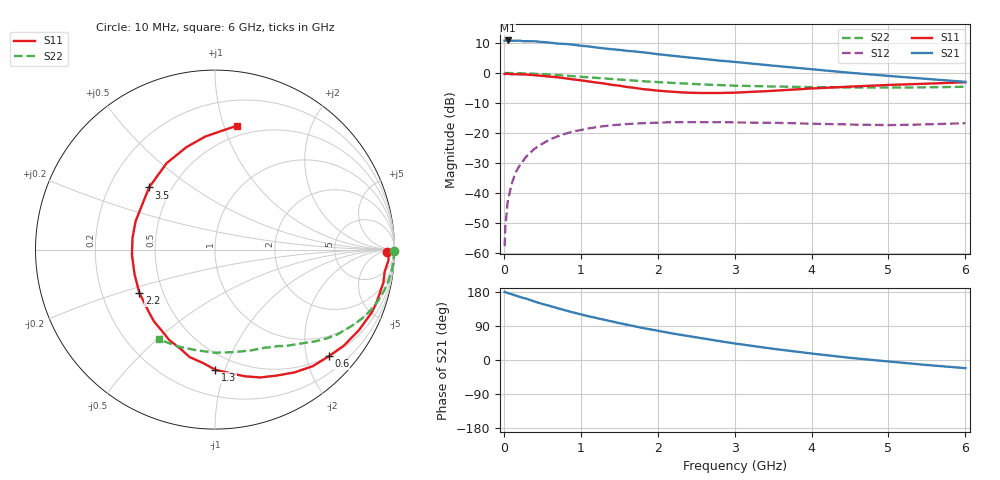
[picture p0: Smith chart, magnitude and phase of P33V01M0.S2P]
! SIEMENS Small Signal Semiconductors
! BFP181
! Si NPN RF Bipolar Junction Transistor in SOT143
! VCE = 3 V  IC = 1 mA
! Common Emitter S-Parameters:  March  1996
# GHz  S  MA  R  50
!  f  S11  S21  S12  S22
! GHz  MAG  ANG  MAG  ANG  MAG  ANG  MAG  ANG
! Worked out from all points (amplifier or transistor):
!   36 points, 10 MHz to 6 GHz, reference 50 ohm
!   highest |S21| = 10.8 dB at 50 MHz (marker M1)
!   |S21| within 3 dB of that: start of sweep to 1.437 GHz
!   unconditionally stable (mu >= 1): 3.116 GHz to end of sweep
!   at 250 MHz: K = 0.09, MSG = 19.9 dB, |S12| = -29.3 dB
!   at 1.4 GHz: K = 0.50, MSG = 12.7 dB, |S12| = -17.4 dB
!   at 6 GHz: K = 1.26, MAG = 3.8 dB, |S12| = -16.7 dB
!   lowest NFmin = 1.30 dB at 450 MHz
!   S11 on the Smith chart (normalised r, x): 10 MHz: 46, -14; 600 MHz: 0.50, -2.44; 1.3 GHz: 0.38, -0.93; 2.2 GHz: 0.37, -0.23; 3.5 GHz: 0.37, +0.35; 6 GHz: 0.41, +1.11
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0.01  0.9608 -0.7  3.449 179.7  0.0013 91.7  0.9986 -0.3
0.02  0.9677 -1.5  3.456 179.3  0.0027 87.7  0.9984 -0.8
0.05  0.9683 -3.5  3.486 176.7  0.0072 88.2  0.9975 -1.7
0.1  0.9533 -7.4  3.436 173.7  0.0139 85.6  0.9966 -3.4
0.2  0.9498 -14.6  3.469 167.1  0.028 80.4  0.9908 -6.8
0.3  0.9408 -21.9  3.389 161.4  0.0418 75.1  0.9823 -10.2
0.4  0.9187 -29.3  3.373 154.3  0.0546 70.9  0.9704 -13.5
0.6  0.869 -43.2  3.2 142.5  0.0781 61.6  0.9419 -19.6
0.8  0.8153 -57.0  3.05 131.0  0.0971 53.6  0.9046 -25.1
0.9  0.7821 -63.8  2.964 125.6  0.1057 49.6  0.8845 -27.7
1.1  0.7247 -76.8  2.774 115.4  0.1191 42.7  0.8465 -32.3
1.3  0.6698 -89.8  2.575 106.4  0.1302 36.3  0.8125 -36.5
1.5  0.6152 -103.3  2.431 97.3  0.1378 30.9  0.7773 -40.2
1.8  0.5398 -123.5  2.216 84.6  0.1454 24.2  0.7312 -45.0
2.2  0.4858 -150.2  1.933 69.7  0.151 16.5  0.6829 -51.1
2.8  0.4642 171.9  1.609 49.9  0.1515 8.0  0.6297 -59.7
3  0.4698 160.3  1.531 43.7  0.1499 5.6  0.6144 -62.7
3.5  0.5049 136.7  1.325 29.6  0.1482 1.8  0.5964 -70.3
4  0.552 119.2  1.156 17.1  0.1429 -1.0  0.581 -79.4
4.5  0.5929 105.5  1.009 5.7  0.1385 -2.4  0.5747 -89.6
5.5  0.6639 86.5  0.797 -13.2  0.1392 0.7  0.5777 -110.8
6  0.7019 79.8  0.712 -21.5  0.1458 1.5  0.5893 -121.8
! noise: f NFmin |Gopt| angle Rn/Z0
0.45  1.3  0.7  18  0.5
0.9  1.4  0.6  39  0.52
1.8  1.85  0.4  81  0.47
